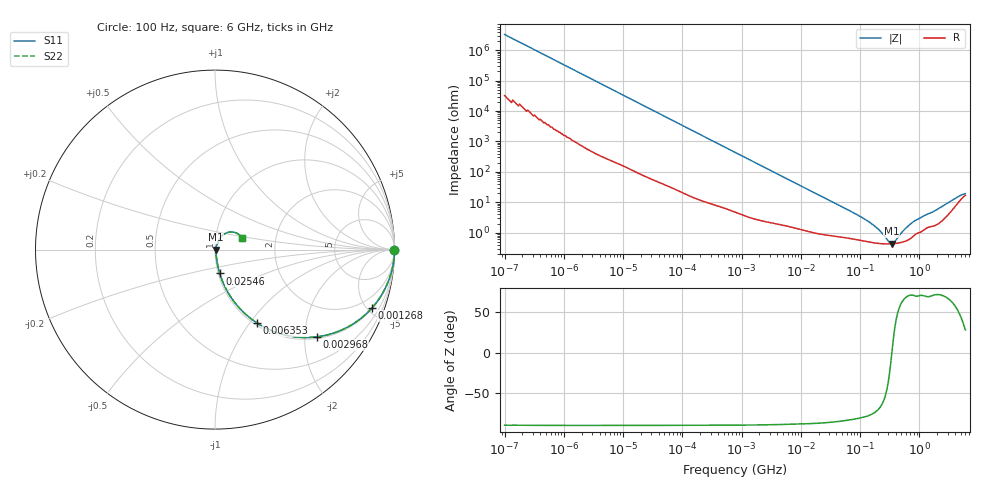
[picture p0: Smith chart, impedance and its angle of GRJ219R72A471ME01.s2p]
!Murata Part Number: GRJ219R72A471ME01
!These Parameters are Measured in Series Mode Connection
!Data Generated on Jun 19, 2026
!  o--ll--o
!Port1  Port2
!  o------o
!Operation Temp=25[degC], DC Bias Voltage=0[V]
!Freq. Start=100[Hz] Stop=6[GHz] 401[Steps]
# Hz S RI R 50
!Freq.(Hz) S11(Real) S11(Imag) S21(Real) S21(Imag) S12(Real) S12(Imag) S22(Real) S22(Imag)
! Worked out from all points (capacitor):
!   401 points, 100 Hz to 6 GHz, reference 50 ohm
!   read as one part in series: C = 484 pF near 109 Hz
!   lowest |Z| = 431 mohm at 341.7 MHz (marker M1)
!   series resonance near 344.2 MHz, so ESL is about 440 pH
!   S11 on the Smith chart (normalised r, x): 100 Hz: open; 1.268 MHz: 1.07, -5.37; 2.968 MHz: 1.04, -2.30; 6.353 MHz: 1.03, -1.09; 25.46 MHz: 1.02, -0.28; 6 GHz: 1.34, +0.18
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100  1 -3.04e-05  3e-07 3.04e-05  3e-07 3.04e-05  1 -3.04e-05
335  1 -0.000101  7e-07 0.000101  7e-07 0.000101  1 -0.000101
2008  1 -0.000604  3e-06 0.000604  3e-06 0.000604  1 -0.000604
40335  0.9998 -0.012  0.00021 0.012  0.00021 0.012  0.9998 -0.012
241822  0.9944 -0.0713  0.00563 0.0713  0.00563 0.0713  0.9944 -0.0713
774597  0.9484 -0.2159  0.0516 0.2159  0.0516 0.2159  0.9484 -0.2159
1267578  0.8751 -0.3245  0.1249 0.3245  0.1249 0.3245  0.8751 -0.3245
1896632  0.7605 -0.4196  0.2395 0.4196  0.2395 0.4196  0.7605 -0.4196
2967816  0.569 -0.4859  0.431 0.4859  0.431 0.4859  0.569 -0.4859
6353432  0.2341 -0.4091  0.7659 0.4091  0.7659 0.4091  0.2341 -0.4091
1.555665e7  0.0565 -0.2095  0.9435 0.2095  0.9435 0.2095  0.0565 -0.2095
2.545746e7  0.0265 -0.1328  0.9735 0.1328  0.9735 0.1328  0.0265 -0.1328
1.395531e8  0.00541 -0.0223  0.9946 0.0223  0.9946 0.0223  0.00541 -0.0223
2.088084e8  0.00452 -0.0114  0.9955 0.0114  0.9955 0.0114  0.00452 -0.0114
3.124326e8  0.00426 -0.00215  0.9957 0.00215  0.9957 0.00215  0.00426 -0.00215
3.417016e8  0.00429 -0.00016  0.9957 0.00016  0.9957 0.00016  0.00429 -0.00016
3.737127e8  0.00435 0.00184  0.9957 -0.00184  0.9957 -0.00184  0.00435 0.00184
5.59173e8  0.00521 0.0114  0.9948 -0.0114  0.9948 -0.0114  0.00521 0.0114
8.000355e8  0.00816 0.0215  0.9918 -0.0215  0.9918 -0.0215  0.00816 0.0215
2.679998e9  0.034 0.0722  0.966 -0.0722  0.966 -0.0722  0.034 0.0722
4.586474e9  0.1007 0.0975  0.8993 -0.0975  0.8993 -0.0975  0.1007 0.0975
6e9  0.15 0.065  0.85 -0.065  0.85 -0.065  0.15 0.065
